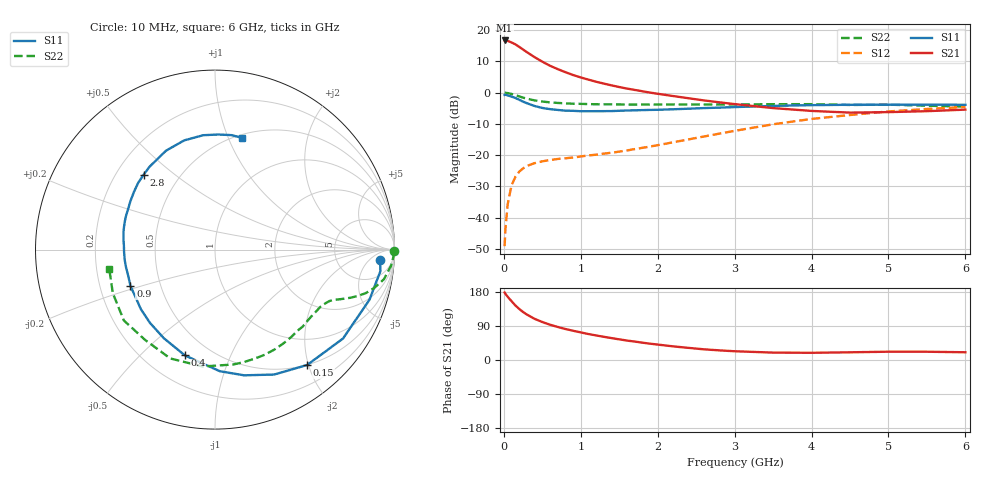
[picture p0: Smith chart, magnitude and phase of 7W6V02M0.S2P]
! Infineon Technologies  Discrete & RF Semiconductors
! BFS17W
! Si NPN RF Bipolar Junction Transistor in SOT323
! VCE = 6 V  IC = 2 mA
! Common Emitter S-Parameters:  August  1999
# GHz  S  MA  R  50
!  f  S11  S21  S12  S22
! GHz  MAG  ANG  MAG  ANG  MAG  ANG  MAG  ANG
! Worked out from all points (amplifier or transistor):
!   36 points, 10 MHz to 6 GHz, reference 50 ohm
!   highest |S21| = 16.7 dB at 10 MHz (marker M1)
!   |S21| within 3 dB of that: start of sweep to 255.6 MHz
!   unconditionally stable (mu >= 1): 838.9 MHz to 2.918 GHz; 4.236 GHz to end of sweep
!   at 250 MHz: K = 0.35, MSG = 19.0 dB, |S12| = -24.2 dB
!   at 1.4 GHz: K = 1.27, MAG = 7.6 dB, |S12| = -19.2 dB
!   at 6 GHz: K = 1.08, MAG = -2.2 dB, |S12| = -4.6 dB
!   S11 on the Smith chart (normalised r, x): 10 MHz: 16, -12; 150 MHz: 0.50, -1.98; 400 MHz: 0.36, -0.69; 900 MHz: 0.33, -0.18; 2.8 GHz: 0.31, +0.39; 6 GHz: 0.53, +1.13
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0.01  0.9208 -3.5  6.854 178.0  0.0035 90.0  0.9998 -0.6
0.02  0.9295 -7.4  6.84 174.8  0.0065 88.2  0.9955 -2.1
0.05  0.9049 -18.0  6.742 166.9  0.0164 80.6  0.9852 -5.2
0.1  0.8683 -34.8  6.365 155.2  0.0329 71.8  0.9561 -9.9
0.15  0.8227 -51.4  5.935 143.9  0.0449 63.1  0.9133 -13.5
0.2  0.7701 -64.7  5.413 134.7  0.0545 57.9  0.8727 -16.2
0.25  0.7188 -77.0  4.906 126.6  0.0615 52.3  0.8335 -18.1
0.3  0.6783 -87.7  4.45 119.9  0.0673 49.4  0.8027 -19.5
0.4  0.6128 -105.9  3.704 108.6  0.0746 44.5  0.7531 -21.5
0.5  0.5701 -120.0  3.137 100.2  0.0798 42.2  0.7221 -22.8
0.6  0.5458 -131.7  2.701 93.1  0.0836 41.3  0.7002 -24.1
0.7  0.5299 -141.2  2.385 87.2  0.087 42.0  0.6859 -25.7
0.9  0.5128 -156.7  1.918 77.2  0.0919 43.5  0.6663 -28.9
1.1  0.5054 -168.8  1.618 68.5  0.0991 46.8  0.6573 -32.8
1.3  0.5068 -178.7  1.398 61.2  0.106 50.6  0.6504 -37.2
1.6  0.519 169.2  1.164 51.3  0.119 56.1  0.6456 -43.9
2.2  0.5431 150.2  0.884 36.0  0.1608 65.1  0.6479 -59.2
2.8  0.5764 133.6  0.702 25.4  0.2209 68.1  0.6474 -75.9
3.5  0.6151 116.3  0.567 19.5  0.3122 65.5  0.6548 -96.0
4.5  0.6408 95.9  0.48 20.3  0.4394 53.6  0.6363 -127.8
5.5  0.6445 81.7  0.506 21.8  0.5484 40.2  0.6189 -156.9
6  0.6399 76.2  0.536 20.4  0.5904 33.7  0.5988 -169.8
